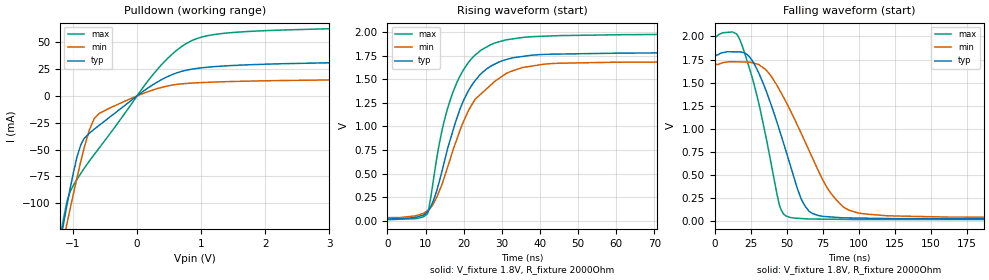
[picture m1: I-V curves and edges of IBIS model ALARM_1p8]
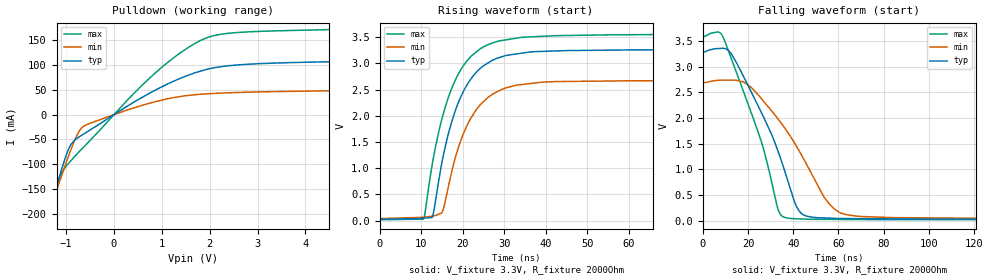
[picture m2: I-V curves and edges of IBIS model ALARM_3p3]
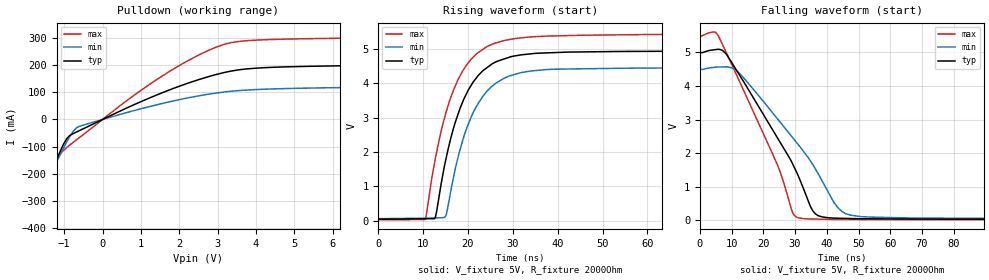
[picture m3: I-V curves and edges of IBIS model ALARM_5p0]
|Texas Instruments Incorporated
| Marketing part#   Digital Voltage Range   Package-type   #pins
|   TMP107   1.8V - 5.0V   SOIC   8
[IBIS Ver]   4.1
[File name]   tmp107.ibs
[File Rev]   1.0
[Date]   05/03/2015
[Source]
| Texas Instruments Incorporated.
| 12500 TI Blvd
| Dallas, TX -75243
[Notes]   Revision History:
| Rev 1.0: 05/03/2015
| - Initial version of the model
| - Model generated from simulations in TISPICE
| - C_comp although listed in numerical order of value are
|   obtained from varying PVT conditions. For PVT conditions for
|   each specific value refer the buffer description under
|   respective [Model]. IBIS model user is responsible for using
|   appropriate C_comp to simulate for Signal Integrity.
| - Warnings regarding combined Non-monotonicity of various models have been
|   reviewd and considered minor and can be ignored.
| - Model names with a trailing _1p8 contain the model for
|   1.8V operation. Model names with a trailing _3p3 contain the model
|   for 3.3V operation.
[Disclaimer]
| This model is designed as an aid for customers of Texas Instruments.
| TI and its licensors and suppliers make no warranties, either expressed
| or implied, with respect to this  model, including the warranties of
| merchantability or fitness for a particular purpose. The model is
| provided solely on an "as is" basis. The entire risk as to its quality
| and performance is with the customer.
[Copyright]
 (C) Copyright 2015 Texas Instruments Incorporated.All rights reserved.
|   Device
[Component]   TMP107
[Manufacturer]   TI
[Package]  | SOIC   8
| variable   typ   min   max
R_pkg   0.1   0.08   0.12
L_pkg   1.0nH   0.8nH   1.2nH
C_pkg   0.2pF   0.16pF   0.24pF
[Pin]  signal_name   model_name   R_pin   L_pin   C_pin
1   V+   POWER   NA   NA   NA
2   R1   NC   NA   NA   NA
3   I/O1   IO1   NA   NA   NA
4   ALERT1  ALARM   NA   NA   NA
5   GND   GND   NA   NA   NA
6   ALERT2  ALARM   NA   NA   NA
7   I/O2   IO2   NA   NA   NA
8   R2   NC   NA   NA   NA
|   Model Selectors
[Model Selector]  IO1
IO1_3p3  IO1 buffer at 3.3V operation.
IO1_5p0  IO1 buffer at 5.0V operation.
IO1_1p8  IO1 buffer at 1.8V operation.
[Model Selector]  IO2
IO2_3p3  IO2 buffer at 3.3V operation.
IO2_5p0  IO2 buffer at 5.0V operation.
IO2_1p8  IO2 buffer at 1.8V operation.
[Model Selector]  ALARM
ALARM_3p3  ALARM buffer at 3.3V operation.
ALARM_5p0  ALARM buffer at 5.0V operation.
ALARM_1p8  ALARM buffer at 1.8V operation.
| Models and submodels in the file (9): ALARM_1p8 (Open_drain), ALARM_3p3 (Open_drain), ALARM_5p0 (Open_drain), IO1_1p8 (I/O), IO1_3p3 (I/O), IO1_5p0 (I/O), IO2_1p8 (I/O), IO2_3p3 (I/O), IO2_5p0 (I/O)
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|   Model
[Model]   ALARM_1p8
Model_type   Open_drain
Polarity   Non-Inverting
Vmeas = 0.9
Vref = 1.8
Cref = 1pF
Rref = 2000
|   typ   min   max
C_comp   1pF   1pF   1pF
[Voltage Range]   1.8   1.7   2
[Temperature Range]   25   125   -55
[Pullup Reference]   1.8   1.7   2
[Pulldown Reference]   0   -0   0
[Power Clamp Reference]   1.8   1.7   2
[GND Clamp Reference]   0   0   0
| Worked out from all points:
|   slope of the pulldown table from 0 to 0.27 V, typ, clamps not added: 23.9 ohm
|   falling waveform, V_fixture 1.8V, R_fixture 2000Ohm: 20-80 % time 22ns typ, 30.8ns min, 16.6ns max; typ from 1.8 V to 0.019 V
|   rising waveform, V_fixture 1.8V, R_fixture 2000Ohm: 20-80 % time 8.93ns typ, 11ns min, 8.02ns max; typ from 0.019 V to 1.8 V
[Pulldown]
|   Voltage   I(typ)   I(min)   I(max)
-1.8V     -345.9mA   -331.3mA   -367.7mA
-1.179V   -129.6mA   -143.5mA   -124.1mA
-1.098V   -103.2mA   -120.4mA   -99.73mA
-1.039V   -84.82mA   -103.7mA   -88.65mA
-941.4mV  -58.1mA    -77.44mA   -78.29mA
-876.6mV  -45.52mA   -60.83mA   -72.22mA
-747mV    -34.96mA   -32.22mA   -60.98mA
-595.8mV  -27.64mA   -16.56mA   -49mA
284.4mV   11.82mA    6.262mA    22.5mA
775.8mV   24.07mA    11.66mA    49.12mA
1.445V    28.24mA    13.39mA    58.92mA
3.6V      31.7mA     15.37mA    63.65mA
[Ramp]
R_load = 2000
|   typ   min   max
dV/dt_r   1.06836/8.91549e-09   0.999769/1.10689e-08   1.19307/8.01726e-09
dV/dt_f   1.06836/2.19556e-08   0.999769/3.06989e-08   1.19307/1.6596e-08
[Falling Waveform]
V_fixture = 1.8V
V_fixture_min = 1.7V
V_fixture_max = 2V
R_fixture = 2000Ohm
C_fixture = 0F
|   Time   V(typ)   V(min)   V(max)
0s        1.8V       1.7V       2V
17.61ns   1.833V     1.724V     1.961V
29.29ns   1.646V     1.701V     1.36V
44.67ns   997.8mV    1.428V     183.9mV
51.94ns   627.4mV    1.214V     37.54mV
59.72ns   247.1mV    958.9mV    24.64mV
66.18ns   94.45mV    737.5mV    19.04mV
83.9ns    37.21mV    233.1mV    16.05mV
100.4ns   28.95mV    82.29mV    13.27mV
500ns     19.32mV    33.53mV    11.52mV
[Rising Waveform]
V_fixture = 1.8V
V_fixture_min = 1.7V
V_fixture_max = 2V
R_fixture = 2000Ohm
C_fixture = 0F
|   Time   V(typ)   V(min)   V(max)
0s        19.32mV    33.53mV    11.52mV
10.47ns   96.6mV     106.4mV    72.83mV
12.9ns    312.5mV    246.8mV    649mV
15.47ns   712.4mV    527.8mV    1.145V
18.21ns   1.087V     864.3mV    1.464V
21.04ns   1.362V     1.149V     1.666V
27.08ns   1.638V     1.437V     1.865V
35.61ns   1.742V     1.624V     1.943V
59.85ns   1.775V     1.68V      1.97V
500ns     1.8V       1.7V       2V
|   Model
[Model]   ALARM_3p3
Model_type   Open_drain
Polarity   Non-Inverting
Vmeas = 1.65
Vref = 3.3
Cref = 1pF
Rref = 2000
|   typ   min   max
C_comp   1pF   1pF   1pF
[Voltage Range]   3.3   2.7   3.6
[Temperature Range]   25   125   -55
[Pullup Reference]   3.3   2.7   3.6
[Pulldown Reference]   -0   0   -0
[Power Clamp Reference]   3.3   2.7   3.6
[GND Clamp Reference]   0   0   0
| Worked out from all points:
|   slope of the pulldown table from 0 to 0.495 V, typ, clamps not added: 16.7 ohm
|   falling waveform, V_fixture 3.3V, R_fixture 2000Ohm: 20-80 % time 18.4ns typ, 22.3ns min, 15.6ns max; typ from 3.3 V to 0.026 V
|   rising waveform, V_fixture 3.3V, R_fixture 2000Ohm: 20-80 % time 7.4ns typ, 7.43ns min, 7.59ns max; typ from 0.026 V to 3.3 V
[Pulldown]
|   Voltage   I(typ)   I(min)   I(max)
-3.3V     -905.6mA   -803.6mA   -1.007A
-1.528V   -258.5mA   -250.1mA   -270.5mA
-1.31V    -182.5mA   -185.6mA   -184.8mA
-1.112V   -116.3mA   -128.5mA   -120.6mA
-933.9mV  -66.35mA   -79.68mA   -96.91mA
-755.7mV  -46.76mA   -38.26mA   -77.77mA
-646.8mV  -39.93mA   -24.31mA   -66.85mA
848.1mV   48.78mA    25.83mA    82.95mA
1.403V    74.07mA    36.92mA    126mA
1.957V    91.93mA    42.16mA    156mA
2.788V    101.8mA    45.35mA    167.2mA
6.6V      111mA      51.08mA    177.1mA
[Ramp]
R_load = 2000
|   typ   min   max
dV/dt_r   1.96439/7.39732e-09   1.59702/7.42838e-09   2.14999/7.5956e-09
dV/dt_f   1.96439/1.83788e-08   1.59702/2.22454e-08   2.14999/1.55879e-08
[Falling Waveform]
V_fixture = 3.3V
V_fixture_min = 2.7V
V_fixture_max = 3.6V
R_fixture = 2000Ohm
C_fixture = 0F
|   Time   V(typ)   V(min)   V(max)
0s        3.3V       2.7V       3.6V
9.105ns   3.364V     2.741V     3.568V
12.89ns   3.238V     2.741V     3.126V
25.7ns    2.126V     2.391V     1.567V
33.37ns   1.339V     1.978V     204.3mV
37.66ns   767.4mV    1.714V     46.72mV
44.24ns   116.4mV    1.229V     30.45mV
56.37ns   46.19mV    304.3mV    22.94mV
68.24ns   37.01mV    85.81mV    20.37mV
500ns     25.95mV    38.11mV    16.66mV
[Rising Waveform]
V_fixture = 3.3V
V_fixture_min = 2.7V
V_fixture_max = 3.6V
R_fixture = 2000Ohm
C_fixture = 0F
|   Time   V(typ)   V(min)   V(max)
0s        25.95mV    38.11mV    16.66mV
10.54ns   45.19mV    63.38mV    27.55mV
12.6ns    58.87mV    85.05mV    1.052V
15.27ns   1.221V     203mV      2.026V
17.57ns   1.946V     1.008V     2.571V
20.49ns   2.518V     1.72V      2.993V
23.28ns   2.832V     2.119V     3.22V
26.21ns   3.016V     2.36V      3.361V
34.02ns   3.193V     2.595V     3.496V
500ns     3.3V       2.7V       3.6V
|   Model
[Model]   ALARM_5p0
Model_type   Open_drain
Polarity   Non-Inverting
Vmeas = 2.5
Vref = 5
Cref = 1pF
Rref = 2000
|   typ   min   max
C_comp   1pF   1pF   1pF
[Voltage Range]   5   4.5   5.5
[Temperature Range]   25   125   -55
[Pullup Reference]   5   4.5   5.5
[Pulldown Reference]   -0   0   -0
[Power Clamp Reference]   5   4.5   5.5
[GND Clamp Reference]   0   0   0
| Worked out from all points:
|   slope of the pulldown table from 0 to 0.75 V, typ, clamps not added: 15 ohm
|   falling waveform, V_fixture 5V, R_fixture 2000Ohm: 20-80 % time 17.7ns typ, 20.5ns min, 15.3ns max; typ from 5 V to 0.036 V
|   rising waveform, V_fixture 5V, R_fixture 2000Ohm: 20-80 % time 7.04ns typ, 6.93ns min, 7.23ns max; typ from 0.036 V to 5 V
[Pulldown]
|   Voltage   I(typ)   I(min)   I(max)
-5V       -1.548A    -1.345A    -1.746A
-2.465V   -600.6mA   -541.1mA   -663.3mA
-1.88V    -388.7mA   -360.4mA   -419.9mA
-1.82V    -367.1mA   -342.2mA   -395.1mA
-1.19V    -145.7mA   -154.6mA   -147.6mA
-935mV    -71.16mA   -83.47mA   -104.1mA
-665mV    -45.28mA   -29.67mA   -73.56mA
1.48V     94.29mA    56.43mA    153.5mA
3.16V     172.9mA    101.2mA    277mA
4.27V     191.5mA    112mA      294.5mA
8.35V     205.3mA    122.9mA    311.4mA
10V       223.5mA    134.4mA    342.1mA
[Ramp]
R_load = 2000
|   typ   min   max
dV/dt_r   2.97845/7.04343e-09   2.66787/6.93753e-09   3.28554/7.23191e-09
dV/dt_f   2.97845/1.77416e-08   2.66787/2.05066e-08   3.28554/1.52609e-08
[Falling Waveform]
V_fixture = 5V
V_fixture_min = 4.5V
V_fixture_max = 5.5V
R_fixture = 2000Ohm
C_fixture = 0F
|   Time   V(typ)   V(min)   V(max)
0s        5V         4.5V       5.5V
5.064ns   5.08V      4.558V     5.581V
8.232ns   4.954V     4.565V     5.007V
24.55ns   2.441V     3.01V      1.631V
29.23ns   1.683V     2.463V     234.4mV
32.47ns   988.9mV    2.078V     58.28mV
36.4ns    198.6mV    1.532V     42.54mV
43.82ns   67.07mV    352.2mV    31.78mV
52.82ns   49.53mV    103.7mV    29.5mV
500ns     35.87mV    53.38mV    24.09mV
[Rising Waveform]
V_fixture = 5V
V_fixture_min = 4.5V
V_fixture_max = 5.5V
R_fixture = 2000Ohm
C_fixture = 0F
|   Time   V(typ)   V(min)   V(max)
0s        35.87mV    53.38mV    24.09mV
10.44ns   50.58mV    67.92mV    26.89mV
12.78ns   114.1mV    76.37mV    1.837V
14.9ns    1.675V     101.4mV    3.049V
17.98ns   3.171V     1.942V     4.154V
19.94ns   3.766V     2.767V     4.579V
21.9ns    4.164V     3.334V     4.86V
26.18ns   4.623V     4.002V     5.179V
33.05ns   4.849V     4.342V     5.344V
500ns     5V         4.5V       5.5V
